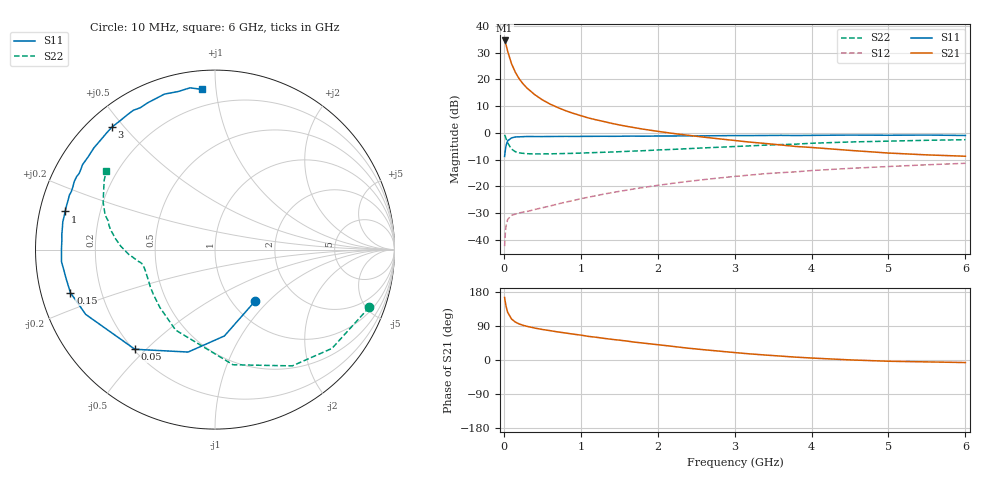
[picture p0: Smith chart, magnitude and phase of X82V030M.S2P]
! SIEMENS Small Signal Semiconductors
! BFP136W
! Si NPN RF Bipolar Junction Transistor in SOT343
! VCE = 2 V  IC = 30 mA
! Common Emitter S-Parameters:  September  1994
# GHz  S  MA  R  50
!  f  S11  S21  S12  S22
! GHz  MAG  ANG  MAG  ANG  MAG  ANG  MAG  ANG
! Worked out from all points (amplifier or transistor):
!   40 points, 10 MHz to 6 GHz, reference 50 ohm
!   highest |S21| = 34.5 dB at 10 MHz (marker M1)
!   |S21| within 3 dB of that: start of sweep to 40.66 MHz
!   unconditionally stable (mu >= 1): 722.2 MHz to 2.811 GHz
!   at 200 MHz: K = 0.43, MSG = 25.0 dB, |S12| = -29.9 dB
!   at 1.5 GHz: K = 1.15, MAG = 10.0 dB, |S12| = -21.8 dB
!   at 6 GHz: K = 0.98, MSG = 1.3 dB, |S12| = -11.3 dB
!   S11 on the Smith chart (normalised r, x): 10 MHz: 1.27, -0.84; 50 MHz: 0.21, -0.46; 150 MHz: 0.09, -0.14; 1 GHz: 0.08, +0.12; 3 GHz: 0.07, +0.46; 6 GHz: 0.10, +0.92
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0.01  0.3633 -51.8  53.12 165.1  0.0077 74.4  0.9177 -20.5
0.02  0.4841 -83.8  48.27 151.6  0.0138 64.0  0.8531 -40.2
0.03  0.5901 -104.7  43.25 140.9  0.0189 54.3  0.7778 -56.4
0.05  0.7125 -128.8  33.26 125.7  0.0243 41.0  0.6494 -81.1
0.1  0.8059 -153.4  19.53 108.2  0.029 29.5  0.4991 -116.1
0.15  0.8405 -163.4  13.5 100.0  0.0305 27.4  0.4454 -133.5
0.2  0.845 -168.9  10.19 95.1  0.0321 27.8  0.4252 -143.6
0.25  0.8516 -173.1  8.235 91.6  0.0333 28.9  0.416 -150.1
0.3  0.858 -175.5  6.897 88.9  0.0341 30.9  0.4093 -154.5
0.4  0.8554 179.9  5.194 84.3  0.0372 35.0  0.4058 -160.1
0.5  0.8548 176.7  4.146 80.6  0.0401 38.2  0.4056 -163.6
0.6  0.8578 174.3  3.456 77.5  0.0432 41.6  0.4071 -165.7
0.8  0.8619 169.7  2.605 71.3  0.051 46.8  0.4129 -168.3
1  0.8617 165.7  2.098 65.7  0.0592 50.3  0.4206 -170.0
1.1  0.8629 163.1  1.903 62.3  0.0631 51.4  0.4251 -170.6
1.5  0.8654 156.3  1.408 52.4  0.0811 54.3  0.4457 -173.1
2.2  0.8754 143.8  0.978 35.8  0.1148 53.3  0.4928 -178.3
3  0.8923 130.0  0.722 19.6  0.1541 48.2  0.5574 173.8
3.2  0.8913 126.6  0.673 16.1  0.1635 46.5  0.5729 171.6
4.5  0.911 108.0  0.472 0.3  0.218 34.8  0.6772 157.0
5.5  0.9119 98.8  0.389 -5.0  0.2541 26.7  0.7283 148.0
6  0.8954 94.5  0.367 -6.7  0.2712 22.1  0.7465 144.2
